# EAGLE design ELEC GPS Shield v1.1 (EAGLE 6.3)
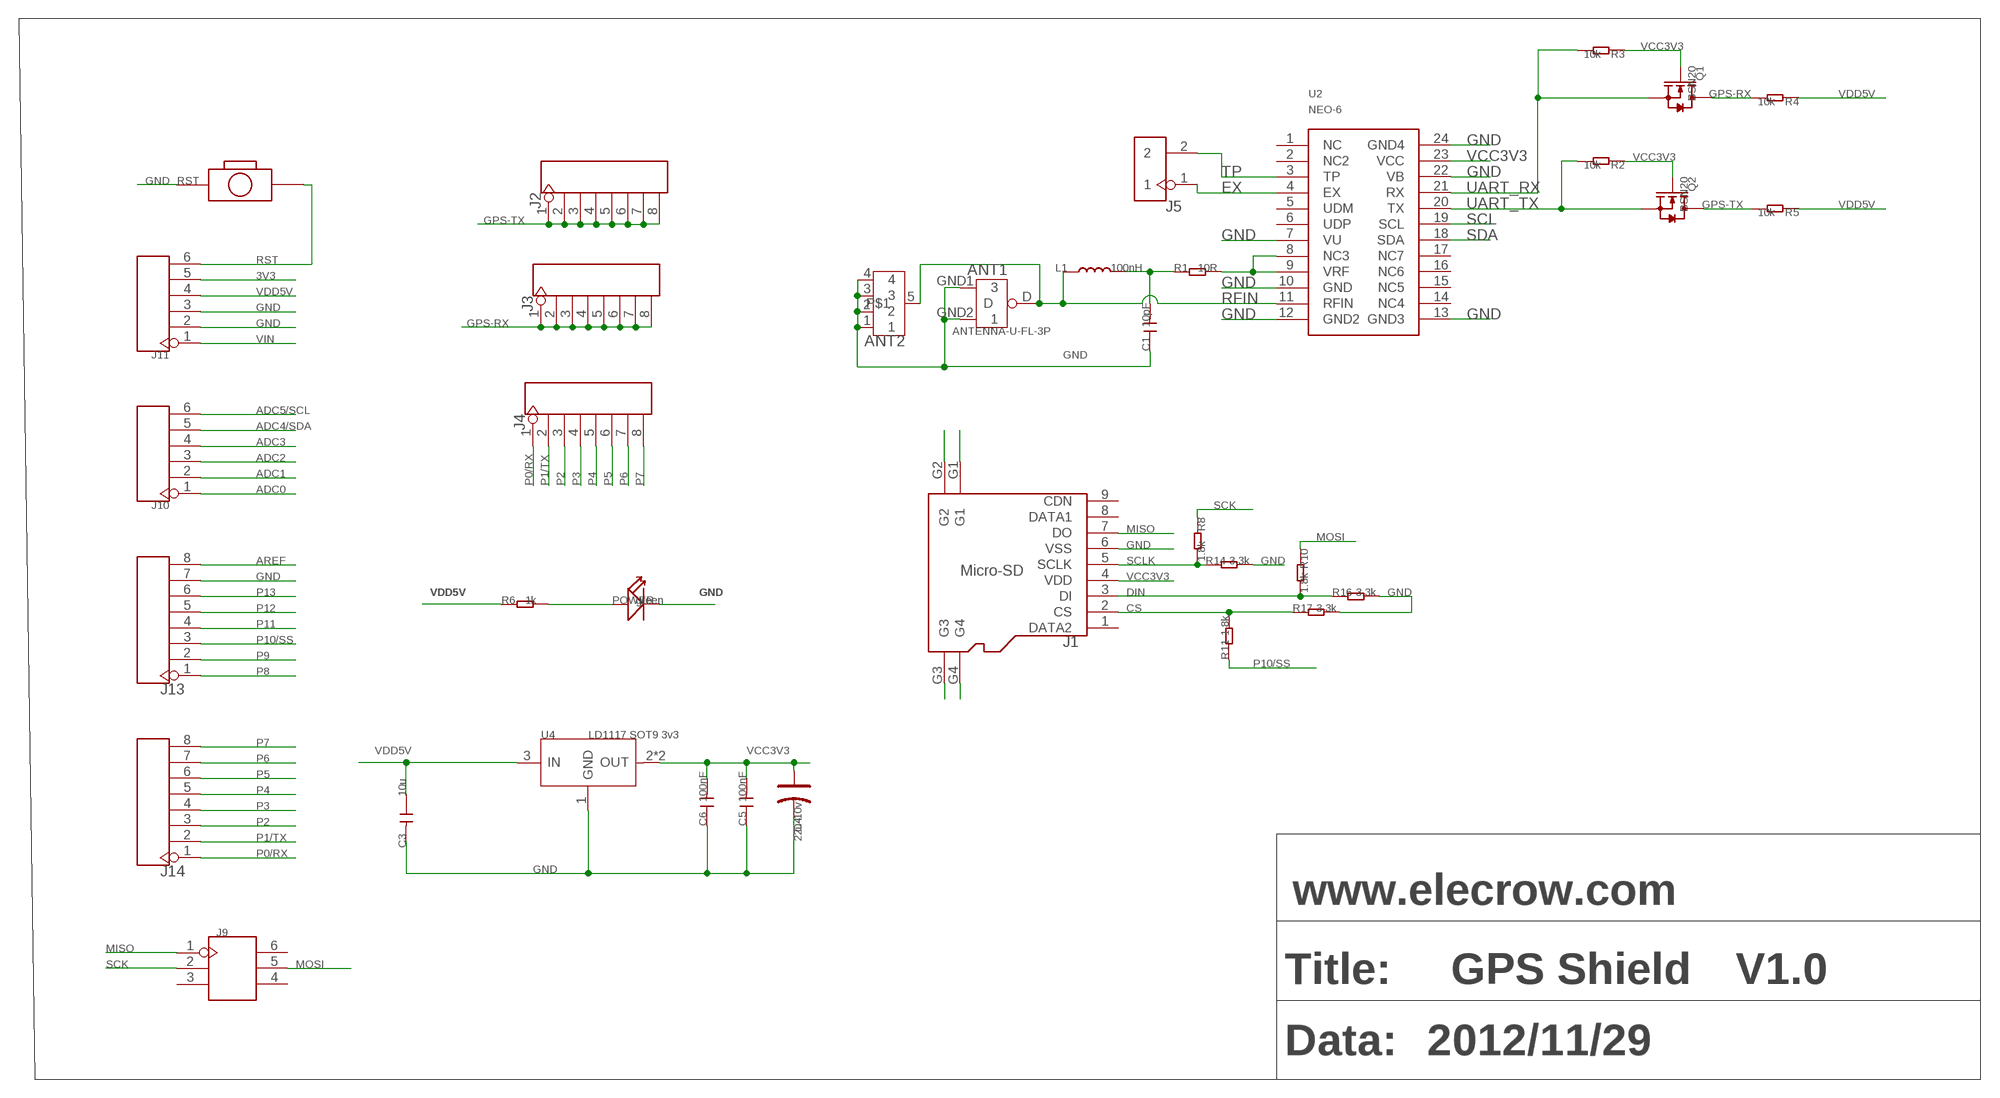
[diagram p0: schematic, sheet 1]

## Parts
ANT1  ANTENNA-U-FL-3P  [3P-U-FL]
ANT2  ANTENNA-SMA-IPX  [SMA-TO-IPX]
C1  10pF  C-0603  [C0603]
C3  10u  C-0805  [C0805]
C4  22u-10v  CAP-AVX-B  [AVX-B]
C5  100nF  C-0603  [C0603]
C6  100nF  C-0603  [C0603]
J1  Micro-SD  HOLDER-MICROSD-9P  [9P-SMD-W/-RING]
J2  HEADER-8P-65/35MIL  [8P-2.54-65/35MIL]
J3  HEADER-8P-65/35MIL  [8P-2.54-65/35MIL]
J4  HEADER-8P-65/35MIL  [8P-2.54-65/35MIL]
J5  HEADER-2P-65/35MIL  [2P-2.54-65/35MIL]
J9  HEADER-2X3P-65/35MIL  [2X3P-2.54-65/35MIL]
J10  HEADER-6P-60/35MIL  [6P-2.54-60/35MIL]
J11  HEADER-6P-60/35MIL  [6P-2.54-60/35MIL]
J13  HEADER-8P-65/35MIL  [8P-2.54-65/35MIL]
J14  HEADER-8P-65/35MIL  [8P-2.54-65/35MIL]
L1  100nH  L'0603'  [L0603]
POWER  green  LED'0603'  [LED-0603]
Q1  BSN20  MOSFET-N'SOT23'  [SOT23]
Q2  BSN20  MOSFET-N'SOT23'  [SOT23]
R1  10R  R-0603  [R0603]
R2  10k  R-0603  [R0603]
R3  10k  R-0603  [R0603]
R4  10k  R-0603  [R0603]
R5  10k  R-0603  [R0603]
R6  1k  R-0603  [R0603]
R8  1.8k  R-0603  [R0603]
R10  1.8k  R-0603  [R0603]
R11  1.8k  R-0603  [R0603]
R14  3.3k  R-0603  [R0603]
R16  3.3k  R-0603  [R0603]
R17  3.3k  R-0603  [R0603]
RST  BOTTON-2P-90D  [2P-7.62X3.56-90D]
U2  NEO-6  [NEO-6]
U4  LD1117 SOT9 3v3  LD1117'SOT89'  [SOT89]

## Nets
3V3: J11.5
ADC0: J10.1
ADC1: J10.2
ADC2: J10.3
ADC3: J10.4
ADC4/SDA: J10.5
ADC5/SCL: J10.6
AREF: J13.8
CS: J1.2(CS) R11.2 R17.1
DIN: J1.3(DI) R10.2 R16.1
EX: J5.1 U2.4(EX)
GND: ANT1.GND1 ANT1.GND2 ANT2.1 ANT2.2 ANT2.3 ANT2.4 C1.1 C3.2 C4.- C5.1 C6.1 J1.6(VSS) J11.2 J11.3 J13.7 POWER.- R14.2 R16.2 R17.2 RST.P$1 U2.7(VU) U2.10(GND) U2.12(GND2) U2.13(GND3) U2.22(VB) U2.24(GND4) U4.1(GND)
GPS-RX: J3.1 J3.2 J3.3 J3.4 J3.5 J3.6 J3.7 J3.8 Q1.3(D) R4.2
GPS-TX: J2.1 J2.2 J2.3 J2.4 J2.5 J2.6 J2.7 J2.8 Q2.3(D) R5.2
MISO: J1.7(DO) J9.1
MOSI: J9.5 R10.1
N$1: POWER.+ R6.2
N$8: R1.2 U2.8(NC3) U2.9(VRF)
N$45: J1.G4
N$46: J1.G3
N$47: J1.G1
N$48: J1.G2
N$61: C1.2 L1.2 R1.1
P0/RX: J4.1 J14.1
P1/TX: J4.2 J14.2
P2: J4.3 J14.3
P3: J4.4 J14.4
P4: J4.5 J14.5
P5: J4.6 J14.6
P6: J4.7 J14.7
P7: J4.8 J14.8
P8: J13.1
P9: J13.2
P10/SS: J13.3 R11.1
P11: J13.4
P12: J13.5
P13: J13.6
RFIN: ANT1.D ANT2.5 L1.1 U2.11(RFIN)
RST: J11.6 RST.P$2
SCK: J9.2 R8.1
SCL: U2.19(SCL)
SCLK: J1.5(SCLK) R8.2 R14.1
SDA: U2.18(SDA)
TP: J5.2 U2.3(TP)
UART_RX: Q1.2(S) R3.2 U2.21(RX)
UART_TX: Q2.2(S) R2.2 U2.20(TX)
VCC3V3: C4.+ C5.2 C6.2 J1.4(VDD) Q1.1(G) Q2.1(G) R2.1 R3.1 U2.23(VCC) U4.2(OUT) U4.4(OUT)
VDD5V: C3.1 J11.4 R4.1 R5.1 R6.1 U4.3(IN)
VIN: J11.1
Unconnected: J1.1(DATA2) J1.8(DATA1) J1.9(CDN) J9.3 J9.4 J9.6 U2.1(NC) U2.2(NC2) U2.5(UDM) U2.6(UDP) U2.14(NC4) U2.15(NC5) U2.16(NC6) U2.17(NC7)

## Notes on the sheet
- www.elecrow.com
- Title: | GPS Shield | V1.0
- Data: | 2012/11/29

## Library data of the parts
ANT1 = Connector:ANTENNA-U-FL-3P
ANT2 = Elecrow_test:ANTENNA-SMA-IPX
C1 C3 C5 C6 = Discrete:C*: Ceramic Capacitors
C4 = Discrete:CAP*: Electrolytic Capacitors,Tantalum Capacitors and Super Capacitors
J1 = Connector:HOLDER-MICROSD-9P
J2-J4 J13 J14 = Connector:HEADER-8P
J5 = Connector:HEADER-2P
J9 = Connector:HEADER-2X3P
J10 J11 = Connector:HEADER-6P
L1 = Discrete:L*
POWER = Discrete:LED*
Q1 Q2 = Discrete:MOSFET-N: IRLL014: http://www.vishay.com/docs/91319/sihll014.pdf
R1-R6 R8 R10 R11 R14 R16 R17 = Discrete:R*
RST = Discrete:BOTTON-2P
U2 = Elecrow_test:NEO-6
U4 = IC:LD1117: Low Drop Fixed And Adjustable Positive Voltage Regulators http://www.datasheetcatalog.org/datasheet/SGSThomsonMicroelectronics/mXuqtqv.pdf

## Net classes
0 default: width 0.152 mm, drill 0.152 mm, clearance 0.152 mm

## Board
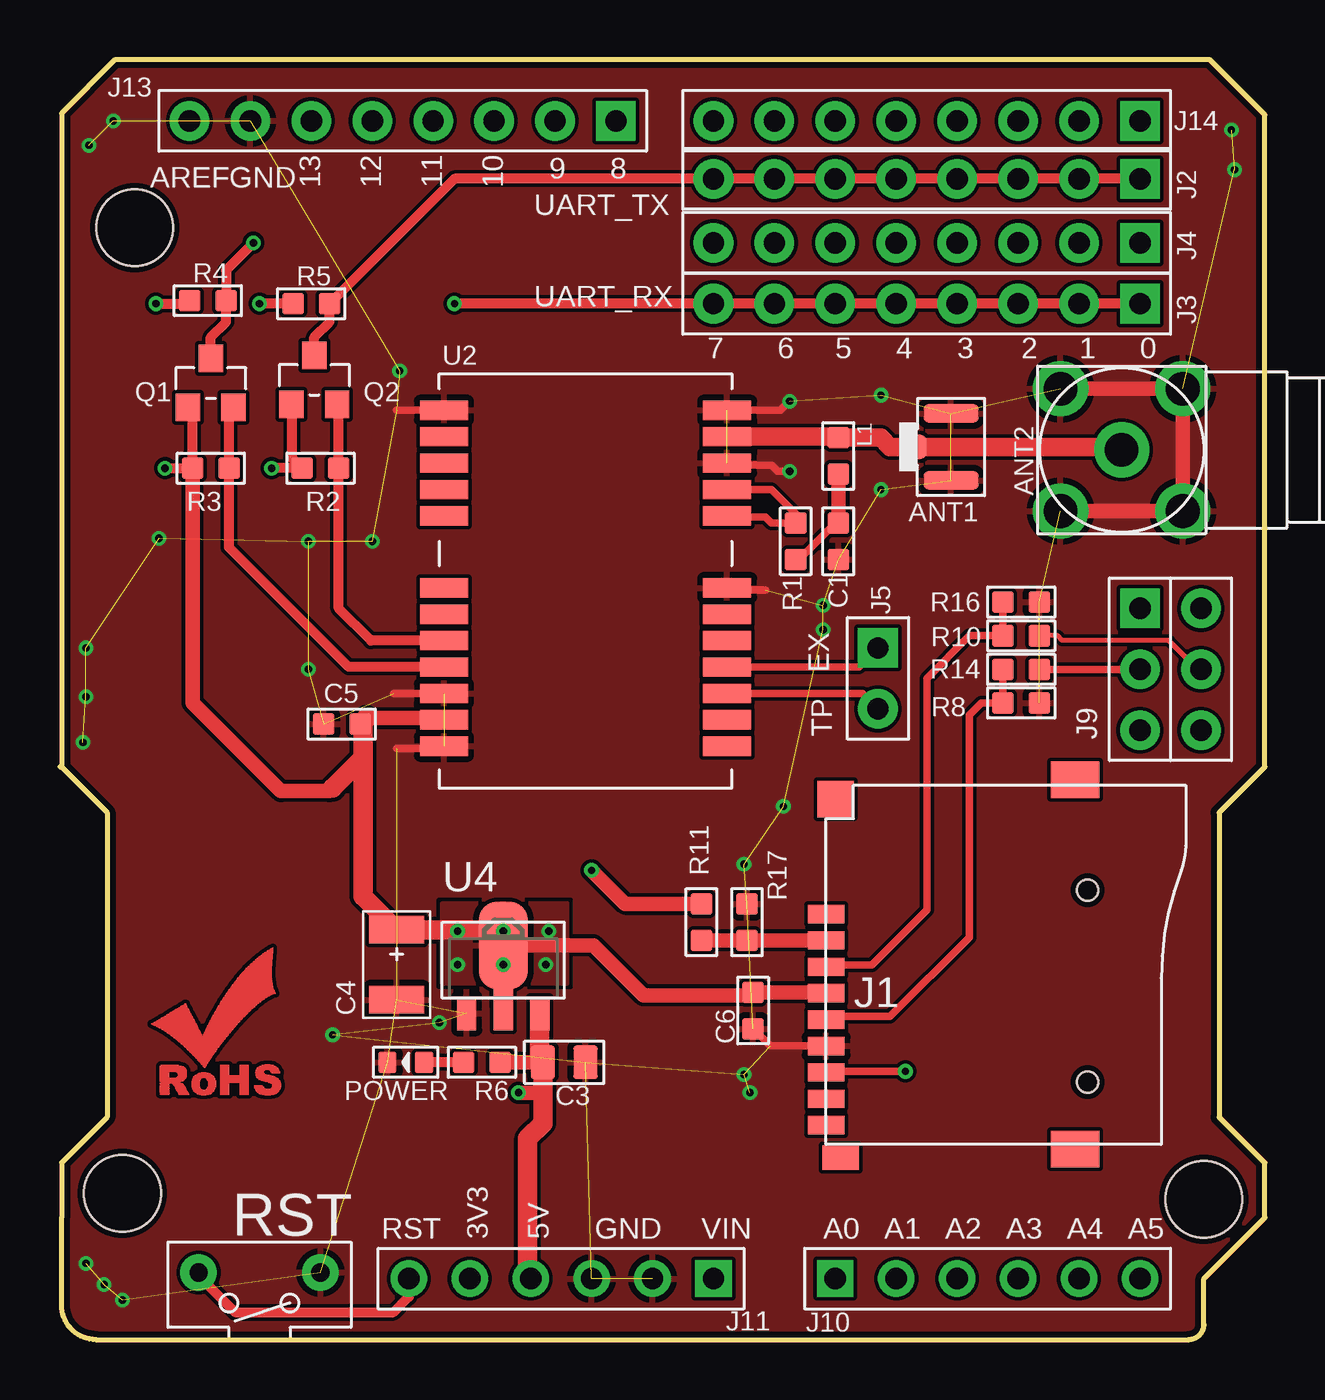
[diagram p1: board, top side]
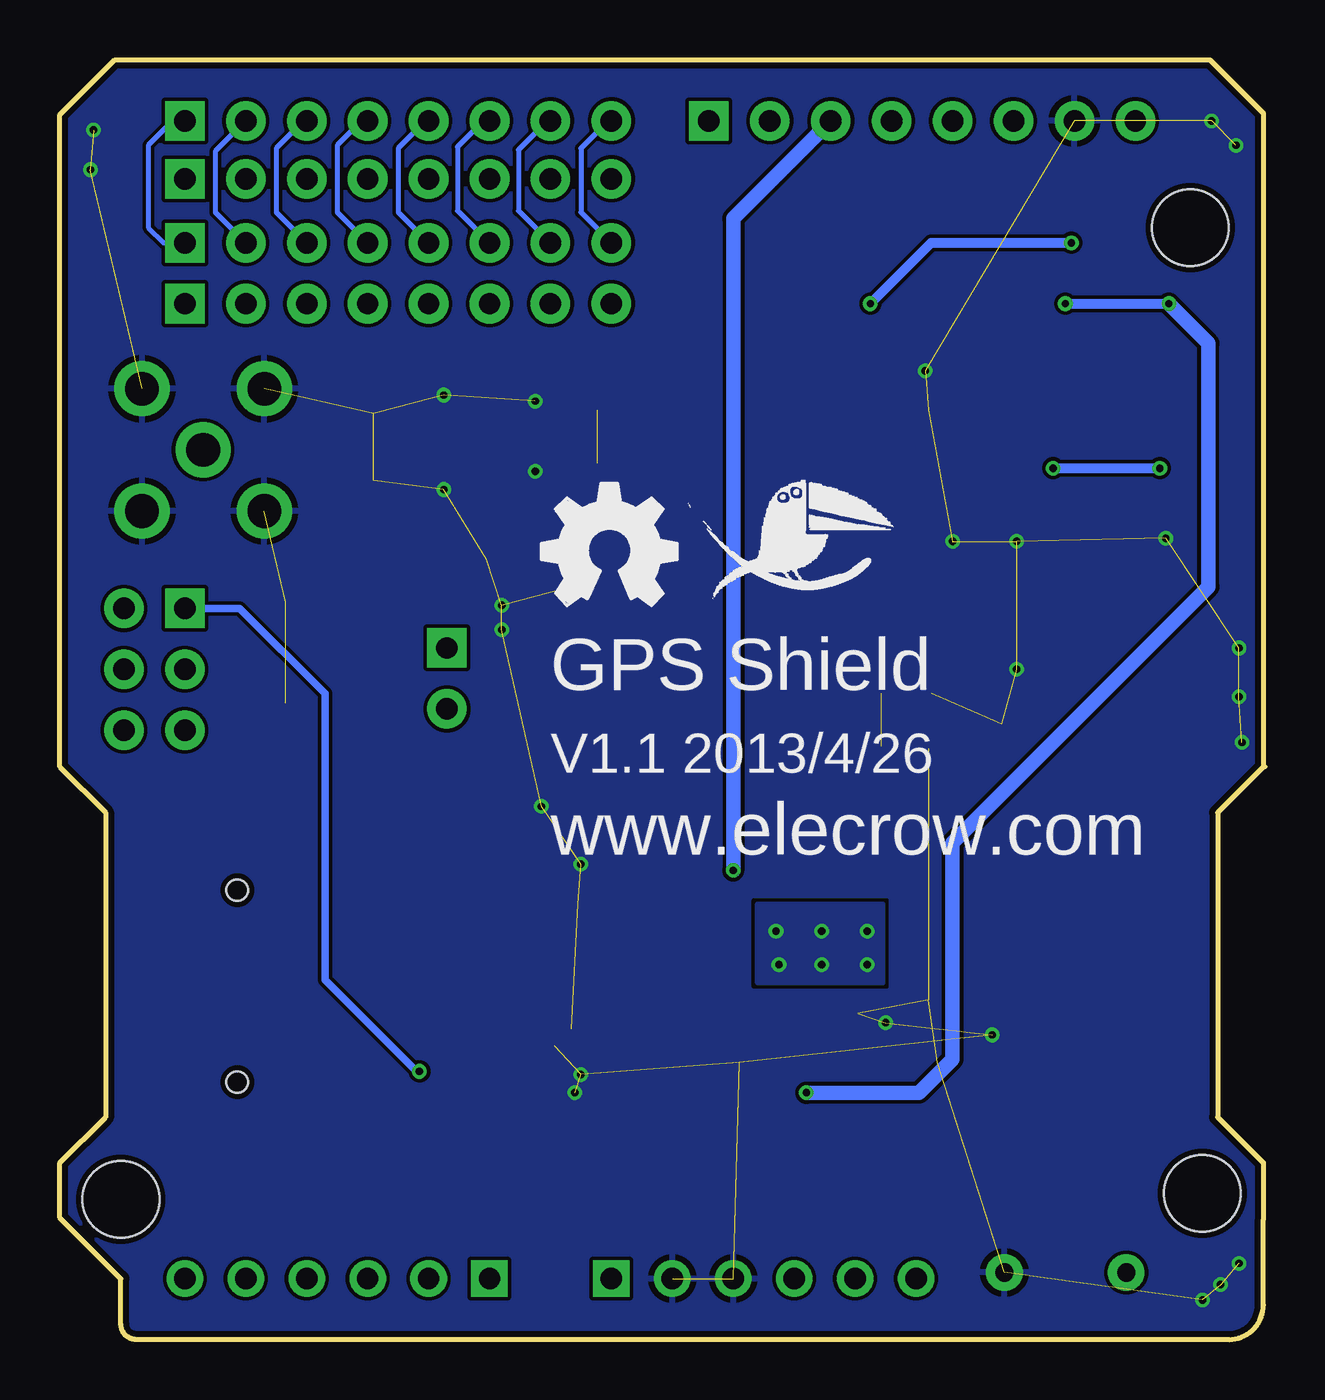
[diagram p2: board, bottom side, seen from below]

Size 50.23 x 53.34 mm. Coordinates in mm from the lower left corner, seen from the top.
Outline: 0.06,23.88 0.06,51.12 2.29,53.34 47.94,53.34 50.23,51.05 50.23,23.88 48.32,21.97 48.32,9.27 50.23,7.37 50.23,5.08 47.69,2.54 47.69,0.64 arc-90 47.05,0 1.5,0 arc-90 0.06,1.44 0.06,5.02
Outline: 0.06,5.08 0.06,7.37 1.97,9.27 1.97,21.97 0.06,23.88
Outline: 0,23.88 0.06,23.88
Copper layers (1*16): Top 0.035mm / dielectric 1.5mm / Bottom 0.035mm
Design rules "SeeedStudio_rule_no_angle_090911 *": minimum track width 6mil, minimum drill 12mil, track to track 6mil, track to pad 6mil, pad to pad 6mil, via to via 6mil, smd to smd 0mil, copper to edge 10mil, drill to drill 10mil, minimum pad ring 10mil, minimum via ring 6mil, stop-mask expansion 2mil, vias tented up to drill 100mil, thermal gap 10mil
Holes 3.2 mm at 47.69,5.84 3.11,46.36 2.6,6.1

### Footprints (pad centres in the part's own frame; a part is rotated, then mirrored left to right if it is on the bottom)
3P-U-FL = smd 1.016 x 1.016: D -1.524,0.127 | smd 2.286 x 0.762: GND1 0,1.524; GND2 0,-1.27
SMA-TO-IPX = drill 1.4 pad 2.3: 1 -2.55,2.55; 2 2.55,2.55; 3 2.55,-2.55; 4 -2.55,-2.55; 5 0,0
C0603 = smd 0.889 x 0.889: 1 -0.762,0; 2 0.762,0
C0805 = smd 1.016 x 1.397: 1 -0.889,0; 2 0.889,0
AVX-B = smd 1.143 x 2.286: + -1.46,0; - 1.46,0
9P-SMD-W/-RING = smd 1.524 x 0.762: 1 0,4.4; 2 0,3.3; 3 0,2.2; 4 0,1.1; 5 0,0; 6 0,-1.1; 7 0,-2.2; 8 0,-3.3; 9 0,-4.4 | smd 1.524 x 1.016: G1 0.6,-5.746 | smd 2.032 x 1.524: G2 10.373,-5.4; G3 10.373,10 | smd 1.524 x 1.524: G4 0.392,9.181 | hole 0.889: 10.9,-2.6; 10.9,5.4
8P-2.54-65/35MIL = drill 0.889 pad 1.651 square: 1 0,8.89 | drill 0.889 pad 1.651: 2 0,6.35; 3 0,3.81; 4 0,1.27; 5 0,-1.27; 6 0,-3.81; 7 0,-6.35; 8 0,-8.89
2P-2.54-65/35MIL = drill 0.889 pad 1.651 square: 1 0,1.27 | drill 0.889 pad 1.651: 2 0,-1.27
2X3P-2.54-65/35MIL = drill 0.889 pad 1.651 square: 1 -1.27,2.54 | drill 0.889 pad 1.651: 2 -1.27,0; 3 -1.27,-2.54; 4 1.27,-2.54; 5 1.27,0; 6 1.27,2.54
6P-2.54-60/35MIL = drill 0.889 pad 1.524 square: 1 0,6.35 | drill 0.889 pad 1.524: 2 0,3.81; 3 0,1.27; 4 0,-1.27; 5 0,-3.81; 6 0,-6.35
L0603 = smd 0.889 x 0.889: 1 -0.762,0; 2 0.762,0
LED-0603 = smd 0.762 x 0.889: + -0.762,0; - 0.762,0
SOT23 = smd 1.016 x 1.143: 1 -0.95,-1.016; 2 0.95,-1.016; 3 0,1.016
R0603 = smd 0.889 x 0.889: 1 -0.762,0; 2 0.762,0
2P-7.62X3.56-90D = drill 0.762 pad 1.524: P$1 0,2.54; P$2 0,-2.54
NEO-6 = smd 2 x 0.8: 1 5.396,-6.507; 2 5.396,-5.407; 3 5.396,-4.307; 4 5.396,-3.207; 5 5.396,-2.107; 6 5.396,-1.007; 7 5.396,0.093; 8 5.396,3.093; 9 5.396,4.193; 10 5.396,5.293; 11 5.396,6.393; 12 5.396,7.493; 13 -6.404,7.493; 14 -6.404,6.393; 15 -6.404,5.293; 16 -6.404,4.193; 17 -6.404,3.093; 18 -6.404,0.093; 19 -6.404,-1.007; 20 -6.404,-2.107; 21 -6.404,-3.207; 22 -6.404,-4.307; 23 -6.404,-5.407; 24 -6.404,-6.507
SOT89 = smd 0.8 x 1.4: 1 -1.524,-1.905; 3 1.524,-1.905 | smd 0.8 x 1.9: 2 0,-1.651 | smd 2.032 x 3.65: 4 0,0.94

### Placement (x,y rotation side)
ANT1  37.15,37.08 0 top
ANT2  44.26,37.08 90 top
C1  32.45,33.27 90 top
C3  21.02,11.56 0 top
C4  14.03,15.62 270 top
C5  11.75,25.65 0 top
C6  28.89,13.72 90 top
J1  31.94,13.34 0 top
J2  36.13,48.39 270 top
J3  36.13,43.18 270 top
J4  36.13,45.72 270 top
J5  34.1,27.56 0 top
J9  46.29,27.94 0 top
J10  38.67,2.54 90 top
J11  20.89,2.54 270 top
J13  14.29,50.8 270 top
J14  36.13,50.8 270 top
L1  32.45,36.83 270 top
POWER  14.41,11.56 180 top
Q1  6.29,39.88 0 top
Q2  10.6,40.01 0 top
R1  30.67,33.27 90 top
R2  10.86,36.32 0 top
R3  6.29,36.32 0 top
R4  6.16,43.31 0 top
R5  10.48,43.18 0 top
R6  17.59,11.56 180 top
R8  40.07,27.94 180 top
R10  40.07,29.34 180 top
R11  26.73,17.4 270 top
R14  40.07,26.54 0 top
R16  40.07,30.73 0 top
R17  28.64,17.4 90 top
RST  8.32,2.79 270 top
U2  22.42,31.24 0 top
U4  18.48,15.49 0 top
U$1  [ROHS_COPPER]  5.91,12.45 0 top
U$2  [OSHW_FILLX200_NOTEXT]  30.16,30.61 0 bottom
U$3  [ELECROW4]  24.19,29.46 0 bottom

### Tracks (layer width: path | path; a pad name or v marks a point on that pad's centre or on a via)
CS
  Top 0.61: R11.2 R17.1 J1.2
DIN
  Top 0.305: R16.1 R10.2 37.91,29.34 36.13,27.56 36.13,17.91 33.85,15.62 32.03,15.62 J1.3
EX
  Top 0.305: U2.4 33.31,28.04 J5.1
GND  (via drill 0.3)  (47 unrouted)
  Top 0.305: U2.7 27.9,31.24 29.4,31.24 | U2.10 27.9,36.45 29.65,36.45 29.91,36.2 v30.42,36.2 | U2.12 30.04,38.74 v30.42,39.12 | U2.13 14.03,38.74 | J1.6 29.61,12.24 C6.1 | U2.22 13.91,26.92 | U2.24 15.91,24.64 14.03,24.64
  Top 0.61: ANT2.1 ANT2.4 ANT2.3 ANT2.2
  other vias: 11.37,12.7 15.81,13.21 28.51,11.05 28.77,10.29 30.16,22.23 28.51,19.81 31.81,29.59 31.81,30.61 34.23,35.43 34.23,39.37 14.16,40.39 13.02,33.27 4.13,33.4 10.35,33.27 10.35,27.94 1.84,2.29 2.6,1.65 1.08,3.18 1.08,28.83 1.08,26.8 0.95,24.89 1.21,49.78 2.22,50.8 48.83,50.42 48.96,48.77
  pour Bottom: -3.62,50.04 -3.62,46.74 -6.92,46.74 -6.92,50.04
  pour Top (rank 6): 0.06,0 50.23,0 50.23,53.34 0.06,53.34 0.06,0.13
  pour Bottom (rank 6): 50.23,0 50.23,53.47 0.06,53.47 0.06,0
GPS-RX  (via drill 0.3)
  Top 0.406: J3.1 J3.2 J3.3 J3.4 J3.5 J3.6 J3.7 J3.8 v16.45,43.18 | Q1.3 6.29,41.78 6.92,42.42 R4.2 6.92,44.58 v8.06,45.72
  Bottom 0.406: v16.45,43.18 13.91,45.72 v8.06,45.72
GPS-TX
  Top 0.406: J2.1 J2.2 J2.3 J2.4 J2.5 J2.6 J2.7 J2.8 16.45,48.39 R5.2 11.24,42.42 10.6,41.78 Q2.3
MISO  (via drill 0.3)
  Top 0.305: J1.7 31.98,11.18 v35.24,11.18
  Bottom 0.305: J9.1 42.74,30.48 39.18,26.92 39.18,14.99 35.37,11.18 v35.24,11.18
MOSI
  Top 0.203: R10.1 41.59,29.34 41.78,29.15 46.23,29.15 47.43,27.94 J9.5
N$1
  Top 0.406: R6.2 POWER.+
N$8
  Top 0.305: U2.8 27.86,34.29 29.4,34.29 29.65,34.04 R1.2 30.67,34.42 29.65,35.43 U2.9
N$61
  Top 0.305: C1.2 32.32,34.04 30.8,32.51 R1.1
  Top 0.61: L1.2 C1.2
P0/RX
  Bottom 0.203: J14.1 45.53,50.8 46.55,49.78 46.55,46.36 45.91,45.72 J4.1
P1/TX
  Bottom 0.203: J14.2 43.75,49.53 43.75,46.99 J4.2
P2
  Bottom 0.203: J14.3 40.07,50.8 41.21,49.66 41.21,46.99 J4.3
P3
  Bottom 0.203: J14.4 37.66,50.8 38.67,49.78 38.67,46.99 J4.4
P4
  Bottom 0.203: J14.5 34.99,50.8 36.13,49.66 36.13,46.99 J4.5
P5
  Bottom 0.203: J14.6 32.58,50.8 33.65,49.72 33.65,47.05 J4.6
P6
  Bottom 0.203: J14.7 29.91,50.8 31.12,49.59 31.12,47.05 J4.7
P7
  Bottom 0.203: J14.8 27.37,50.8 28.51,49.66 28.51,46.99 J4.8
P10/SS  (via drill 0.3)
  Top 0.61: v22.16,19.56 23.56,18.16 R11.1
  Bottom 0.61: J13.3 22.16,46.74 v22.16,19.56
RFIN
  Top 0.61: U2.11 27.85,37.59
  Top 0.762: U2.11 32.45,37.64 | L1.1 34.23,37.59 34.61,37.21 ANT1.D 44.13,37.21 ANT2.5
  Top 0.813: 32.45,37.64 L1.1
RST
  Top 0.406: RST.P$2 5.78,2.67 7.3,1.14 13.91,1.14 14.54,1.78 J11.6
SCK
  Top 0.305: J9.2 R8.1
SCLK
  Top 0.305: R8.2 R14.1 38.42,26.54 37.91,26.04 37.91,16.76 34.61,13.46 32.07,13.46 J1.5
TP
  Top 0.305: U2.3 33.45,26.94 J5.2
UART_RX
  Top 0.406: U2.21 12.03,28.04 7.05,33.02 R3.2 7.05,38.67 Q1.2
UART_TX
  Top 0.406: U2.20 12.97,29.14 11.62,30.48 R2.2 11.62,38.92 Q2.2
VCC3V3  (via drill 0.3)
  Top 0.406: v8.83,36.32 R2.1 9.65,36.76 Q2.1 | v4.38,36.32 R3.1 5.52,38.67 Q1.1
  Top 0.61: 12.76,25.91 15.94,25.91 U2.23 | U4.4 22.24,16.43 24.32,14.35 28.77,14.35 C6.2 31.9,14.48 J1.4 | 11.37,22.99 11.24,22.86 9.21,22.86 5.52,26.54 R3.1
  Top 0.813: U4.2 v18.48,15.62 U4.4 17.83,17.08 C4.+ 12.64,18.48 12.64,24.26 | 11.37,22.99 12.64,24.26 | 12.64,24.26 12.64,25.53 C5.2 12.76,25.91
  Bottom 0.406: v8.83,36.32 v4.38,36.32
  other vias: 16.57,15.62 20.26,15.62 20.38,17.02 16.57,17.02 18.48,17.02
  pour Top: 15.94,14.86 16.07,14.86 21.15,14.86 21.15,18.16 15.94,18.16
  pour Bottom: 15.94,14.86 21.15,14.86 21.15,17.53 21.15,18.16 15.94,18.16
VDD5V  (via drill 0.3)
  Top 0.406: R5.1 v8.32,43.18 | v4,43.18 5.27,43.18 R4.1
  Top 0.61: R6.1 C3.1 | v19.11,10.29 20.13,10.29
  Top 0.813: J11.4 19.49,2.67 19.49,8.38 20.13,9.02 20.13,10.29 C3.1 20,11.68 U4.3
  Bottom 0.406: v8.32,43.18 v4,43.18
  Bottom 0.61: v4,43.18 2.35,41.53 2.35,31.37 13.02,20.7 13.02,11.68 14.41,10.29 v19.11,10.29

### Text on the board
tPlace: AREF | GND | 13 | 12 | 11 | 10 | 9 | 8 | UART_TX | UART_RX | 7 | 6 | 5 | 4 | 3 | 2 | 1 | 0 | EX | TP | RST | 3V3 | 5V | GND | VIN | A0 | A1 | A2 | A3 | A4 | A5
bPlace: GPS Shield | V1.1 2013/4/26 | www.elecrow.com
